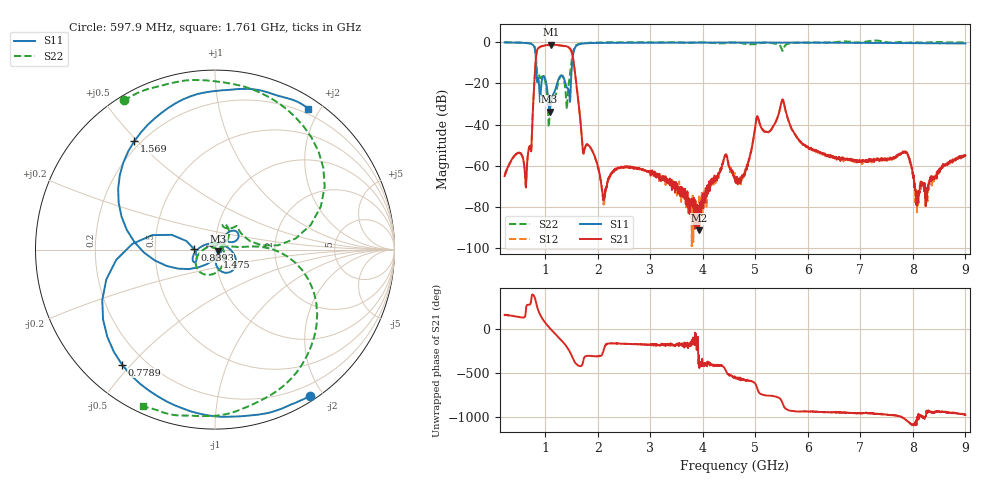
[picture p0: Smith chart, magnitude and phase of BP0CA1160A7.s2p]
!Agilent Technologies,E8358A,US41080443,A.07.50.56
!Agilent E8358A: A.07.50.56
!Date: Thursday, November 09, 2017 08:41:01
!Correction: S11(Full 2 Port(1,2))
!S21(Full 2 Port(1,2))
!S12(Full 2 Port(1,2))
!S22(Full 2 Port(1,2))
!S2P File: Measurements: S11, S21, S12, S22:
# Hz S  dB  R 50
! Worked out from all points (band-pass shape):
!   1601 points, 225 MHz to 9 GHz, reference 50 ohm
!   highest |S21| = -1.20 dB at 1.113 GHz (marker M1); lowest = -91.4 dB at 3.927 GHz (marker M2)
!   |S21| within 3 dB of the highest: 840.3 MHz to 1.496 GHz (655.7 MHz wide, 56.1 % of centre)
!   lowest |S11| = -33.8 dB at 1.081 GHz (marker M3), VSWR 1.04, Z = 51.8 - j1.05 ohm
!   |S11| at or under -10 dB: 824.8 MHz to 1.512 GHz (686.8 MHz wide, 58.8 % of centre)
!   |S22| runs from -41.3 to 0.9 dB; largest |S21 - S12| = 0.016
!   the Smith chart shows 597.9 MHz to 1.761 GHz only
!   S11 on the Smith chart (normalised r, x): 597.9 MHz: 0.06, -1.84; 778.9 MHz: 0.12, -0.47; 839.2 MHz: 0.79, +0.00; 1.475 GHz: 1.02, -0.08; 1.569 GHz: 0.18, +0.49; 1.761 GHz: 0.13, +1.85
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2.25e8  -0.06 -15.5  -65.09 158.0  -64.72 158.3  -0.00 163.2
5.979375e8  -0.25 -56.9  -59.67 129.9  -60.14 130.4  -0.23 121.5
7.789219e8  -1.68 -128.9  -25.11 19.9  -25.30 19.9  -1.28 58.8
8.3925e8  -18.83 179.7  -4.29 -97.9  -4.44 -97.7  -13.89 13.3
9.653906e8  -16.36 -50.2  -1.63 96.8  -1.77 97.0  -16.63 63.3
1.080562e9  -33.79 -29.7  -1.24 11.6  -1.38 11.7  -34.88 139.8
1.113469e9  -28.29 18.1  -1.20 -9.7  -1.37 -9.6  -27.98 127.6
1.354781e9  -17.53 23.8  -1.67 -162.6  -1.82 -162.4  -18.40 -151.4
1.475438e9  -27.71 -71.4  -3.18 89.7  -3.32 89.7  -14.50 5.1
1.568672e9  -2.47 126.7  -15.40 -24.4  -15.56 -23.9  -1.90 -52.8
1.689328e9  -0.69 71.7  -44.29 -59.8  -44.44 -59.4  -0.55 -100.0
1.760625e9  -0.51 56.5  -50.79 47.0  -51.01 47.2  -0.35 -114.6
2.117109e9  -0.22 20.6  -76.56 129.8  -78.09 121.8  -0.08 -143.5
3.153656e9  -0.18 -21.7  -65.31 176.8  -65.96 -177.6  -0.01 -167.3
3.926953e9  -0.17 -37.5  -91.43 59.9  -74.16 -62.0  0.00 -175.0
4.6125e9  -0.06 -45.6  -66.30 162.5  -66.41 165.8  -0.01 173.7
5.511938e9  -0.20 -53.2  -27.97 -116.4  -28.03 -116.4  -3.99 155.0
6.076828e9  -0.14 -59.0  -52.20 143.4  -52.17 142.0  -0.14 146.0
7.541156e9  -0.36 -84.5  -56.61 103.8  -56.76 101.5  -0.10 110.1
7.881188e9  -0.38 -93.5  -53.94 38.8  -53.83 37.9  -0.10 104.4
8.084109e9  -0.39 -99.5  -73.84 83.0  -73.42 46.0  0.01 106.9
9e9  -0.49 -128.6  -55.11 103.6  -55.26 105.8  -0.04 97.2
